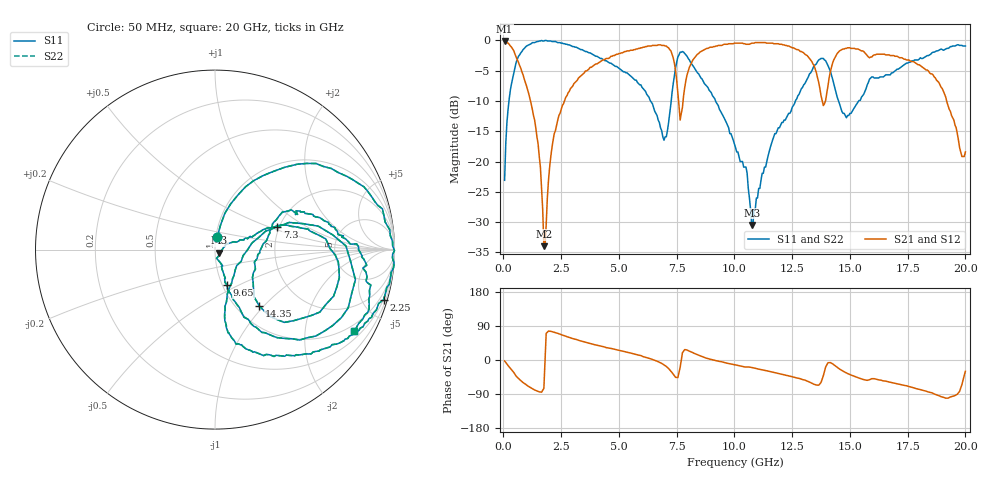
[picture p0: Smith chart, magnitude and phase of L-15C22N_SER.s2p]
# MHZ S MA R 50
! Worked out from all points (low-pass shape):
!   400 points, 50 MHz to 20 GHz, reference 50 ohm
!   highest |S21| = -0.09 dB at 50 MHz (marker M1); lowest = -34.0 dB at 1.75 GHz (marker M2)
!   |S21| within 3 dB of the highest: 8.227 GHz to 13.27 GHz (5.045 GHz wide, 46.9 % of centre); 14.32 GHz to 17.35 GHz (3.027 GHz wide, 19.1 % of centre)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
!   lowest |S11| = -30.5 dB at 10.75 GHz (marker M3), VSWR 1.06, Z = 52.4 - j1.87 ohm
!   |S11| at or under -10 dB: 6.369 GHz to 7.263 GHz (893.9 MHz wide, 13.1 % of centre); 9.184 GHz to 12.64 GHz (3.457 GHz wide, 31.7 % of centre); 14.51 GHz to 15.38 GHz (872.1 MHz wide, 5.84 % of centre)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
!   |S22| runs from -30.5 to 0.0 dB; largest |S21 - S12| = 0
!   S11 on the Smith chart (normalised r, x): 50 MHz: 1.02, +0.14; 2.25 GHz: 0.49, -6.86; 7.3 GHz: 1.95, +0.58; 9.65 GHz: 1.05, -0.44; 14.35 GHz: 1.26, -0.94; 20 GHz: 0.74, -3.55
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50  0.07 79.8  0.99 -2.4  0.99 -2.4  0.07 79.8
200  0.27 71.0  0.95 -14.6  0.95 -14.6  0.27 71.0
500  0.6 49.8  0.77 -37.8  0.77 -37.8  0.6 49.8
1350  0.96 9.3  0.22 -79.1  0.22 -79.1  0.96 9.3
1750  0.99 -2.7  0.02 -74.7  0.02 -74.7  0.99 -2.7
2250  0.98 -16.5  0.18 72.2  0.18 72.2  0.98 -16.5
3400  0.84 -40.2  0.52 49.5  0.52 49.5  0.84 -40.2
6700  0.22 -67.9  0.92 -4.5  0.92 -4.5  0.22 -67.9
7050  0.16 -12.2  0.9 -17.0  0.9 -17.0  0.16 -12.2
7300  0.37 20.1  0.77 -33.3  0.77 -33.3  0.37 20.1
7650  0.8 -12.1  0.22 -19.6  0.22 -19.6  0.8 -12.1
7950  0.74 -40.6  0.52 26.3  0.52 26.3  0.74 -40.6
9650  0.21 -71.4  0.93 -8.0  0.93 -8.0  0.21 -71.4
10050  0.13 -70.0  0.95 -12.9  0.95 -12.9  0.13 -70.0
10750  0.03 -36.5  0.95 -19.7  0.95 -19.7  0.03 -36.5
13350  0.56 9.5  0.67 -61.3  0.67 -61.3  0.56 9.5
13850  0.71 -21.4  0.29 -41.3  0.29 -41.3  0.71 -21.4
14350  0.4 -51.9  0.72 -14.7  0.72 -14.7  0.4 -51.9
14850  0.23 -17.5  0.86 -34.3  0.86 -34.3  0.23 -17.5
16700  0.52 24.0  0.76 -58.1  0.76 -58.1  0.52 24.0
18600  0.8 1.1  0.52 -88.0  0.52 -88.0  0.8 1.1
20000  0.9 -30.3  0.12 -29.8  0.12 -29.8  0.9 -30.3
